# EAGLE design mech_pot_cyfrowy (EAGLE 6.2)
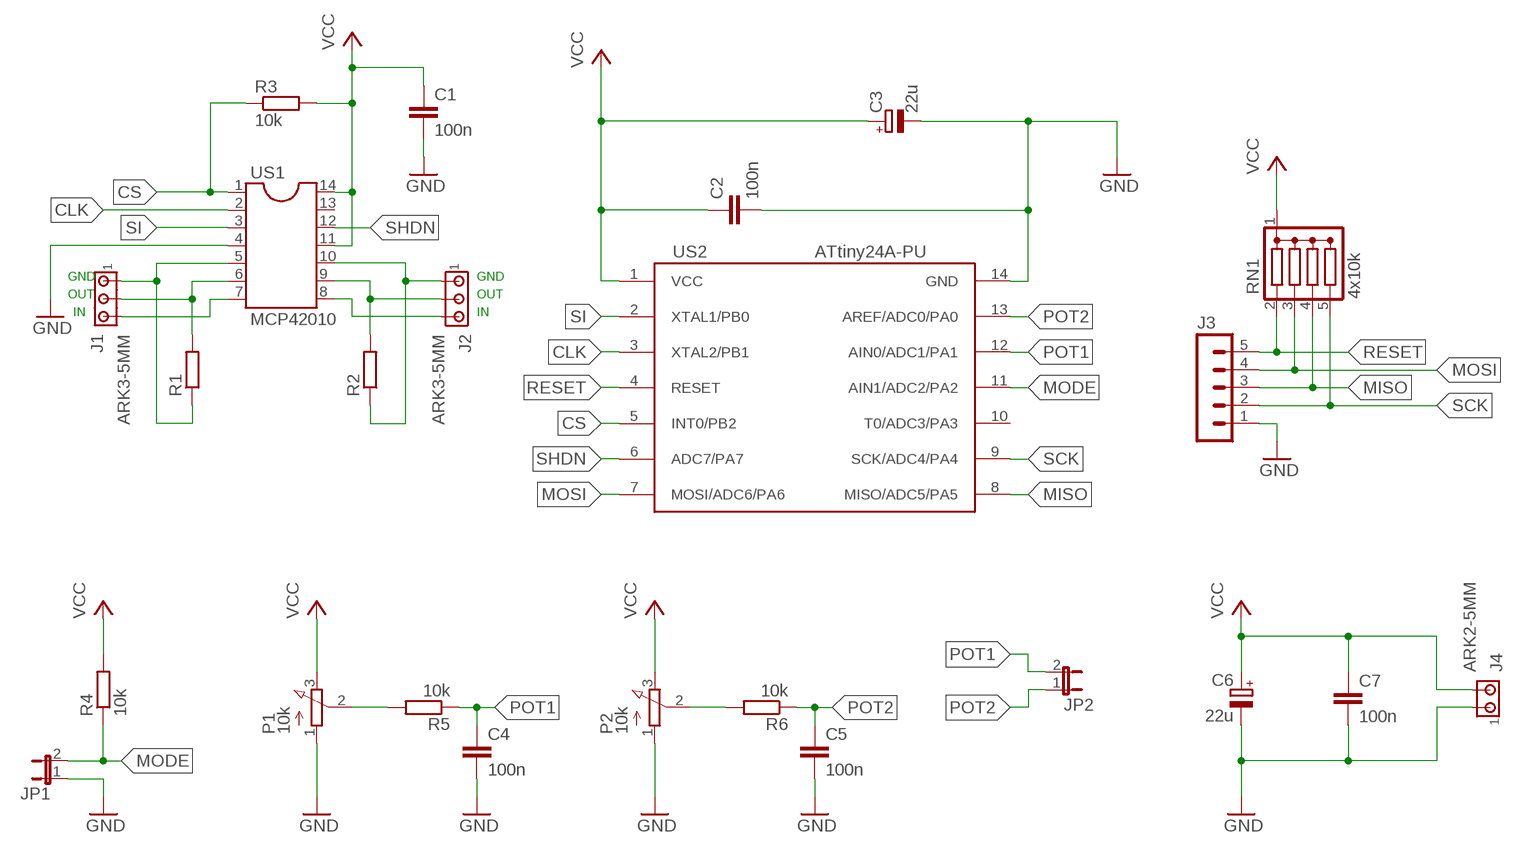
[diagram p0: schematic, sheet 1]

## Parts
C1  100n  C-EU050-025X075  [C050-025X075]
C2  100n  C-EU050-025X075  [C050-025X075]
C3  22u  CPOL-EUE2.5-5  [E2,5-5]
C4  100n  C-EU050-025X075  [C050-025X075]
C5  100n  C-EU050-025X075  [C050-025X075]
C6  22u  CPOL-EUE2.5-5  [E2,5-5]
C7  100n  C-EU050-025X075  [C050-025X075]
J1  ARK3-5MM  [3PIN-5MM]
J2  ARK3-5MM  [3PIN-5MM]
J3  MA05-1  [MA05-1]
J4  ARK2-5MM  [2PIN-5MM]
JP1  JP1E  [JP1]
JP2  JP1E  [JP1]
P1  10k  3RP/1610N  [POT_POJEDYNCZY]
P2  10k  3RP/1610N  [POT_POJEDYNCZY]
R1  R-EU_0207/7  [0207/7]
R2  R-EU_0207/7  [0207/7]
R3  10k  R-EU_0207/7  [0207/7]
R4  10k  R-EU_0207/7  [0207/7]
R5  10k  R-EU_0207/7  [0207/7]
R6  10k  R-EU_0207/7  [0207/7]
RN1  4x10k  DRAB_REZ_1X4  [RN-5]
US1  MCP42010  DIL14  [DIL14]
US2  ATtiny24A-PU  ATTINY24/44/84-PU  [DIL14]

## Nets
CLK: US1.2 US2.3(XTAL2/PB1)
CS: R3.1 US1.1 US2.5(INT0/PB2)
GND: C1.2 C2.2 C3.- C4.2 C5.2 C6.- C7.2 J3.1 J4.P$1 JP1.1 P1.1(A) P2.1(A) US1.4 US2.14(GND)
MISO: J3.3 RN1.4 US2.8(MISO/ADC5/PA5)
MODE: JP1.2 R4.1 US2.11(AIN1/ADC2/PA2)
MOSI: J3.4 RN1.3 US2.7(MOSI/ADC6/PA6)
N$1: J1.P$1 R1.1 US1.5
N$2: J1.P$2 R1.2 US1.6
N$3: J1.P$3 US1.7
N$4: J2.P$1 R2.1 US1.10
N$5: J2.P$2 R2.2 US1.9
N$6: J2.P$3 US1.8
N$7: P1.2(S) R5.2
N$8: P2.2(S) R6.2
POT1: C4.1 JP2.2 R5.1 US2.12(AIN0/ADC1/PA1)
POT2: C5.1 JP2.1 R6.1 US2.13(AREF/ADC0/PA0)
RESET: J3.5 RN1.2 US2.4(RESET)
SCK: J3.2 RN1.5 US2.9(SCK/ADC4/PA4)
SHDN: US1.12 US2.6(ADC7/PA7)
SI: US1.3 US2.2(XTAL1/PB0)
VCC: C1.1 C2.1 C3.+ C6.+ C7.1 J4.P$2 P1.3(E) P2.3(E) R3.2 R4.2 RN1.1(C) US1.11 US1.14 US2.1(VCC)
Unconnected: US1.13 US2.10(T0/ADC3/PA3)

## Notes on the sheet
- GND | GND
- OUT | OUT
- IN | IN

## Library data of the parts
C1 C2 C4 C5 C7 = rcl:C-EU: CAPACITOR, European symbol
C3 C6 = rcl:CPOL-EU: POLARIZED CAPACITOR, European symbol
J1 J2 = zlacza_futrzak:ARK3: ARK 3 Raster 5mm i 3,5mm
J3 = zlacza_futrzak:MA05-1: PIN HEADER; OC_FARNELL: unknown; OC_NEWARK: unknown
J4 = zlacza_futrzak:ARK2: ARK 2
JP1 JP2 = jumper:JP1E: JUMPER
P1 P2 = inne_futrzak:3RP/1610N: 16mm Potentiometer one level Source: http://www.alphapotentiometers.net/html/16mm_pot_2.html
R1-R6 = rcl:R-EU_: RESISTOR, European symbol
RN1 = inne_futrzak:DRAB_REZ_1X4
US1 = ic-package:DIL14: Dual In Line / Socket
US2 = scalaki_futrzak:ATTINY24/44/84

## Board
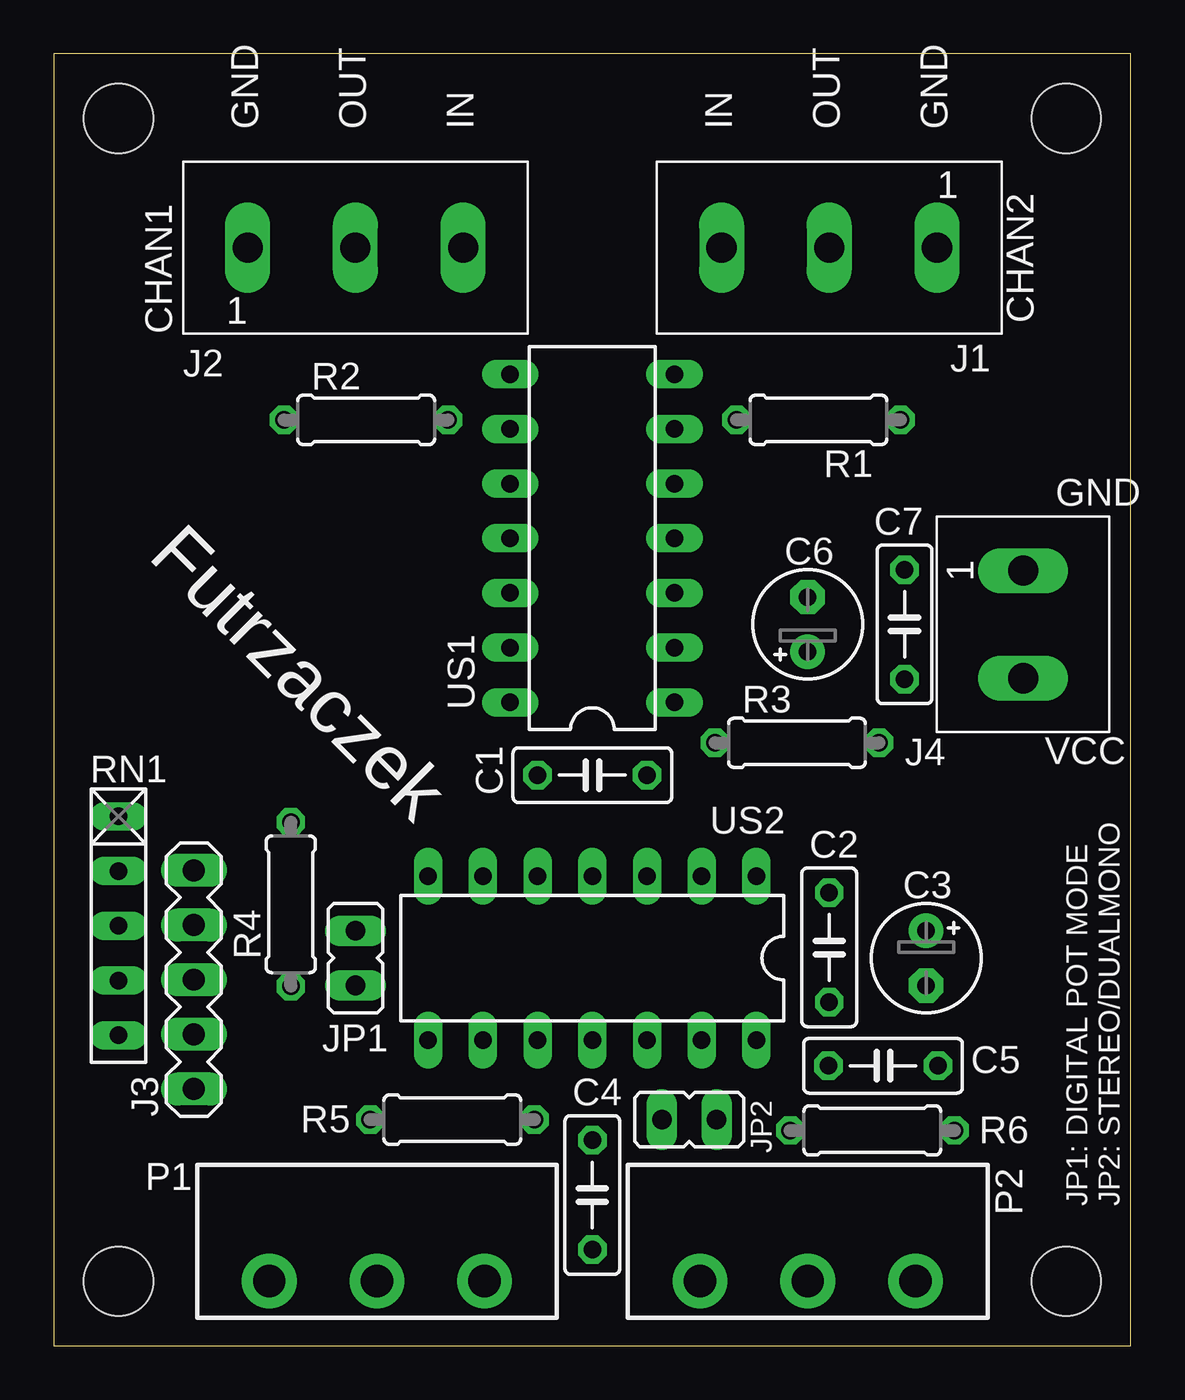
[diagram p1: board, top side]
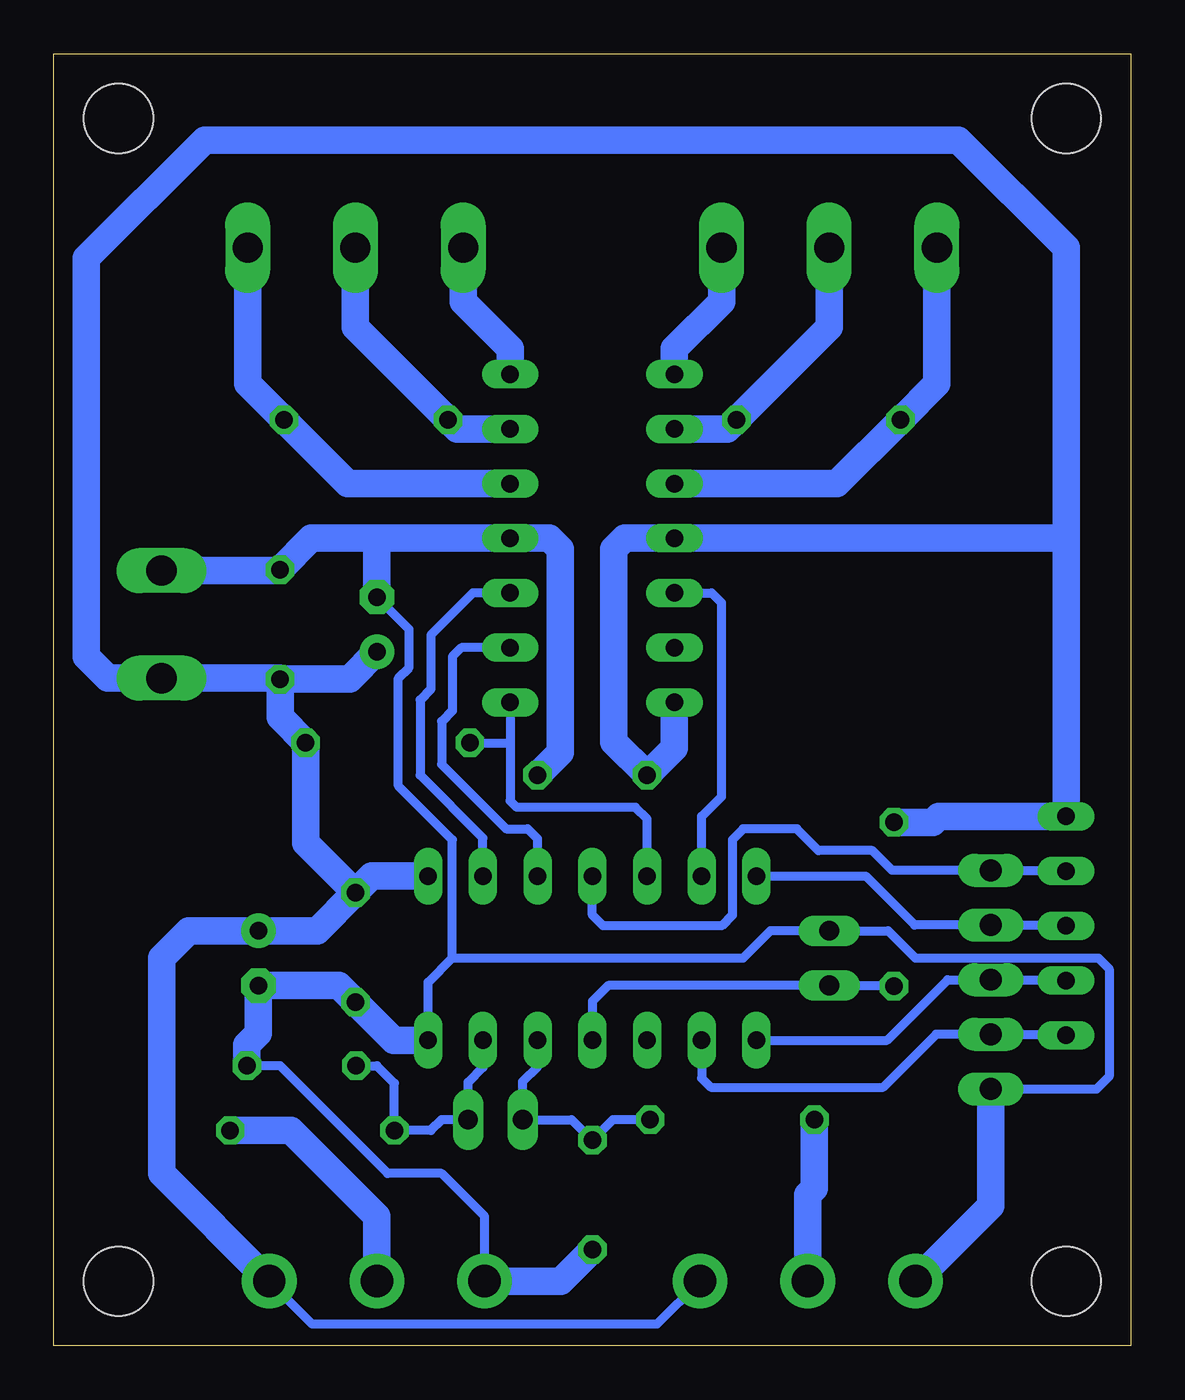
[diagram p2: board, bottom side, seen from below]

Size 50 x 60 mm. Coordinates in mm from the lower left corner, seen from the top.
Outline: 0,0 50,0 50,60 0,60 0,0
Copper layers (1*16): Top 0.035mm / dielectric 1.5mm / Bottom 0.035mm
Design rules: minimum track width 10mil, minimum drill 24mil, track to track 8mil, track to pad 8mil, pad to pad 8mil, via to via 8mil, smd to smd 8mil, copper to edge 40mil, drill to drill 8mil, minimum pad ring 10mil, minimum via ring 8mil, stop-mask expansion 4mil, vias tented up to drill 0mil, thermal gap 10mil
Holes 3.2 mm at 3,3 3,57 47,3 47,57

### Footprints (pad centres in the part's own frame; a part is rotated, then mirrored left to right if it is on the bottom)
C050-025X075 = drill 0.813 octagon: 1 -2.54,0; 2 2.54,0
E2,5-5 = drill 0.813 pad 1.6: + -1.27,0 | drill 0.813 pad 1.6 octagon: - 1.27,0
3PIN-5MM = drill 1.4 long: P$1 -5,0; P$2 0,0; P$3 5,0
MA05-1 = drill 1.016 long: 1 -5.08,0; 2 -2.54,0; 3 0,0; 4 2.54,0; 5 5.08,0
2PIN-5MM = drill 1.4 long: P$1 -2.5,0; P$2 2.5,0
JP1 = drill 0.914 long: 1 0,-1.27; 2 0,1.27
POT_POJEDYNCZY = drill 1.5 pad 2.54: 1 -5,0; 2 0,0; 3 5,0
0207/7 = drill 0.813 octagon: 1 -3.81,0; 2 3.81,0
RN-5 = drill 0.813 long: 1 -5.08,0; 2 -2.54,0; 3 0,0; 4 2.54,0; 5 5.08,0
DIL14 = drill 0.813 long: 1 -7.62,-3.81; 2 -5.08,-3.81; 3 -2.54,-3.81; 4 0,-3.81; 5 2.54,-3.81; 6 5.08,-3.81; 7 7.62,-3.81; 8 7.62,3.81; 9 5.08,3.81; 10 2.54,3.81; 11 0,3.81; 12 -2.54,3.81; 13 -5.08,3.81; 14 -7.62,3.81

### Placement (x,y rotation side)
C1  25,26.5 0 top
C2  36,18.5 270 top
C3  40.5,18 270 top
C4  25,7 270 top
C5  38.5,13 0 top
C6  35,33.5 90 top
C7  39.5,33.5 90 top
J1  36,51 180 top
J2  14,51 0 top
J3  6.5,17 90 top
J4  45,33.5 270 top
JP1  14,18 180 top
JP2  29.5,10.5 90 top
P1  15,3 0 top
P2  35,3 0 top
R1  35.5,43 180 top
R2  14.5,43 0 top
R3  34.5,28 0 top
R4  11,20.5 90 top
R5  18.5,10.5 180 top
R6  38,10 0 top
RN1  3,19.5 270 top
US1  25,37.5 90 top
US2  25,18 180 top

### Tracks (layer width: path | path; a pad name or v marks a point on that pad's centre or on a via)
CLK
  Bottom 0.406: US1.2 31.08,32.42 31.5,32 31.5,29.5 32,29 32,27 29,24 28,24 27.54,23.54 US2.3
CS
  Bottom 0.406: US2.5 22.46,24.46 23,25 28.5,25 28.81,25.31 28.81,28 | US1.1 28.81,28 | R3.1 28.81,28
GND
  Bottom 0.406: US2.14 32.62,16.88 31.5,18 | 31.5,18 18,18 16.73,19.27 JP1.1 11.27,19.27 10,18 1.5,18 1,17.5 1,12.5 1.58,11.92 J3.1 | P2.1 30,6 32,8 34.5,8 39.5,13 C5.2 | 31.5,18 31.5,23.5 34,26 34,31 33.5,31.5 33.5,33.27 C6.-
  Bottom 1.27: J4.P$1 39.54,36 C7.2 38.04,37.5 35,37.5 | 35,37.5 US1.4 27,37.5 26.5,37 26.5,27.54 C1.2 | C6.- 35,37.5 | US2.14 34.23,14.19 C2.2 36.77,16.73 C3.- 40.5,14.5 41.04,13.96 C5.2 | J3.1 6.5,6.5 P1.1 | P2.1 26.46,3 C4.2
MISO
  Bottom 0.406: US2.8 11.31,14.19 8.5,17 J3.3 2.54,17 RN1.4
MODE
  Bottom 0.406: R4.1 11.04,16.73 JP1.2 24.27,16.73 25,16 US2.11
MOSI
  Bottom 0.406: US2.7 12.31,21.81 10.04,19.54 J3.4 2.54,19.54 RN1.3
N$1
  Bottom 1.27: US1.5 36.35,40.04 R1.1 41,44.69 J1.P$1
N$2
  Bottom 1.27: US1.6 31.27,42.58 R1.2 36,47.31 J1.P$2
N$3
  Bottom 1.27: US1.7 28.81,46.31 31,48.5 J1.P$3
N$4
  Bottom 1.27: US1.10 13.65,40.04 R2.1 9,44.69 J2.P$1
N$5
  Bottom 1.27: US1.9 18.73,42.58 R2.2 14,47.31 J2.P$2
N$6
  Bottom 1.27: US1.8 21.19,46.31 19,48.5 J2.P$3
N$7
  Bottom 1.27: R5.2 14.69,7.31 15,7 P1.2
N$8
  Bottom 1.27: P2.2 35,6 39,10 R6.2
POT1
  Bottom 0.406: US2.12 27.54,12.96 28.23,12.27 JP2.2 25.96,10.5 C4.1 24.04,10.5 R5.1
POT2
  Bottom 0.406: US2.13 30.08,12.92 30.77,12.23 JP2.1 32,10.5 32.5,10 R6.1 34.19,12.19 35,13 C5.1
RESET
  Bottom 0.406: RN1.2 2.54,22.08 J3.5 11.08,22.08 12,23 14.5,23 15.5,24 18,24 18.5,23.5 18.5,20 19,19.5 24.5,19.5 25,20 US2.4
SCK
  Bottom 0.406: US2.9 19.92,12.42 19.5,12 11.5,12 9.04,14.46 J3.2 2.54,14.46 RN1.5
SHDN
  Bottom 0.406: US2.6 19.92,24.58 19,25.5 19,34.5 19.46,34.96 US1.12
SI
  Bottom 0.406: US1.3 30.54,34.96 32.5,33 32.5,30.5 33,30 33,26.5 30.08,23.58 US2.2
VCC
  Bottom 0.406: P1.3 22,1 38,1 P2.3
  Bottom 1.27: C7.1 39.54,31 J4.P$2 47.5,31 48.5,32 48.5,50.5 43,56 8,56 3,51 3,37.5 | C7.1 36.27,30.96 C6.+ | C7.1 39.5,29.19 R3.2 38.31,23.35 C2.1 | US1.14 21.19,27.77 C1.1 24,28.04 24,37 23.5,37.5 US1.11 3,37.5 | R4.2 9.19,24.31 8.92,24.58 RN1.1 3,37.5 | C2.1 37.77,19.27 C3.+ 43.73,19.27 45,18 45,8 P2.3 | US2.1 35.23,21.81 C2.1

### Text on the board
tPlace: GND | OUT | IN | IN | OUT | GND | CHAN2 | CHAN1 | GND | VCC | Futrzaczek | JP1: DIGITAL POT MODE | JP2: STEREO/DUALMONO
